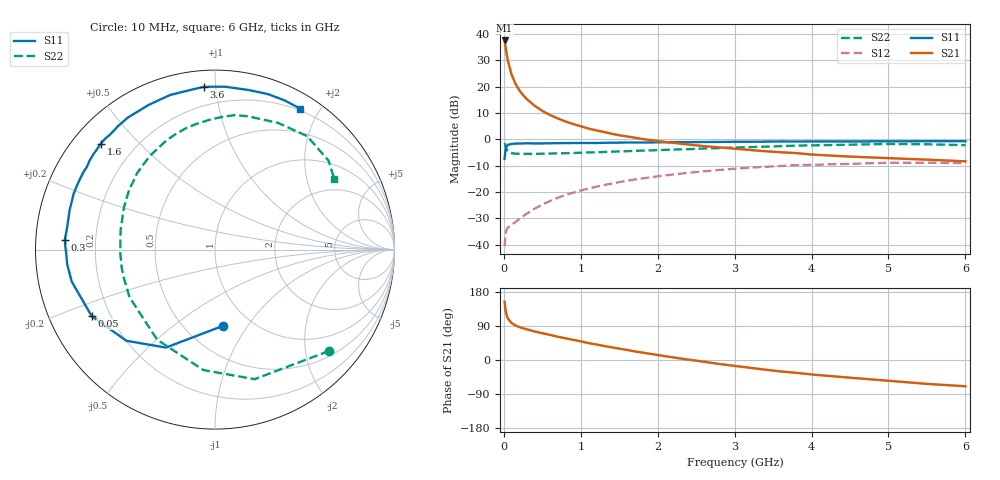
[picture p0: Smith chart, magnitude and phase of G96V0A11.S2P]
! SIEMENS Small Signal Semiconductors
! BFG235
! Si NPN RF Bipolar Junction Transistor in SOT223
! VCE = 6 V  IC = 110 mA
! Common Emitter S-Parameters:  July  1994
# GHz  S  MA  R  50
!  f  S11  S21  S12  S22
! GHz  MAG  ANG  MAG  ANG  MAG  ANG  MAG  ANG
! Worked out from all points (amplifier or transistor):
!   40 points, 10 MHz to 6 GHz, reference 50 ohm
!   highest |S21| = 37.6 dB at 10 MHz (marker M1)
!   |S21| within 3 dB of that: start of sweep to 25.1 MHz
!   unconditionally stable (mu >= 1): 462 MHz to 1.387 GHz
!   at 200 MHz: K = 0.78, MSG = 24.5 dB, |S12| = -30.3 dB
!   at 1.5 GHz: K = 0.99, MSG = 8.9 dB, |S12| = -16.3 dB
!   at 6 GHz: K = 0.90, MSG = 0.4 dB, |S12| = -9.1 dB
!   S11 on the Smith chart (normalised r, x): 10 MHz: 0.75, -0.78; 50 MHz: 0.13, -0.25; 300 MHz: 0.09, +0.03; 1.6 GHz: 0.08, +0.39; 3.6 GHz: 0.09, +0.93; 6 GHz: 0.18, +1.76
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0.01  0.4265 -83.7  75.43 153.6  0.0093 64.6  0.8503 -41.6
0.02  0.6105 -116.6  60.09 135.0  0.0152 50.0  0.7549 -73.0
0.03  0.7085 -134.2  47.68 123.1  0.018 42.1  0.6743 -95.5
0.05  0.7807 -151.7  32.06 110.1  0.0208 34.3  0.5964 -122.7
0.1  0.8178 -167.4  17.04 97.5  0.0239 36.0  0.5452 -150.8
0.15  0.8276 -174.3  11.44 91.2  0.0267 41.1  0.5319 -162.5
0.2  0.8284 -177.9  8.564 87.1  0.0305 45.4  0.5299 -169.1
0.25  0.8341 178.8  6.905 83.6  0.0345 48.9  0.527 -173.6
0.3  0.8387 176.4  5.762 80.9  0.0387 51.6  0.5279 -177.4
0.4  0.8332 171.7  4.337 75.3  0.048 55.1  0.5278 177.4
0.5  0.8348 168.1  3.463 70.5  0.0575 56.7  0.5314 173.2
0.6  0.8394 164.9  2.891 66.3  0.0671 57.0  0.5354 169.3
0.7  0.8419 161.4  2.489 61.5  0.0772 56.7  0.5397 165.9
0.8  0.8467 158.5  2.181 57.4  0.0871 55.7  0.5426 162.7
1.1  0.8507 149.5  1.597 44.7  0.1159 51.5  0.5614 153.8
1.6  0.868 137.1  1.133 26.6  0.1624 41.7  0.5926 140.1
2.2  0.8812 123.5  0.854 6.8  0.2142 28.8  0.637 124.2
3.2  0.8969 101.9  0.625 -20.6  0.288 5.6  0.7088 98.0
3.6  0.9089 93.9  0.567 -30.2  0.3109 -4.4  0.7408 86.8
4.5  0.9087 78.2  0.468 -46.7  0.3412 -24.3  0.7884 63.6
5.5  0.9174 64.9  0.41 -63.0  0.36 -46.5  0.8036 38.1
6  0.9177 58.8  0.381 -69.3  0.3499 -54.8  0.7729 30.7
